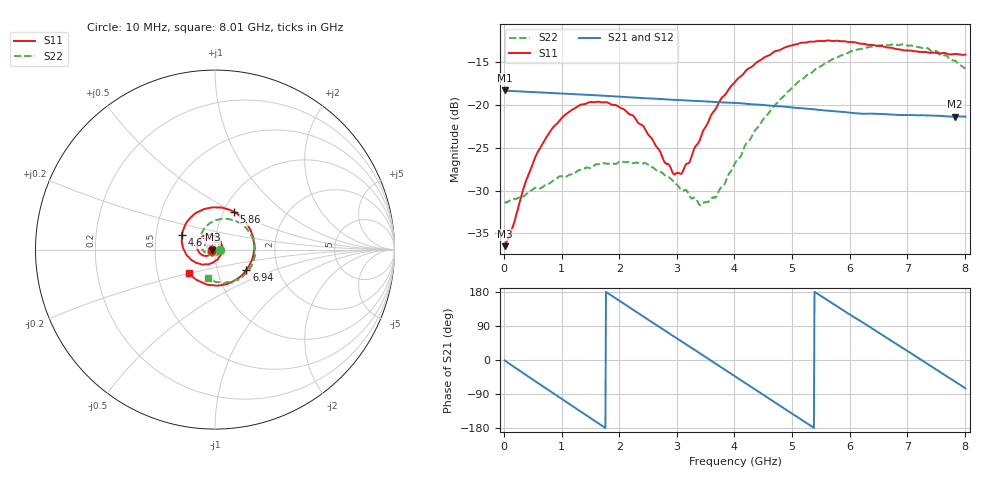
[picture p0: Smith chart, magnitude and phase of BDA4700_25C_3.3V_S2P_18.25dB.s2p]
!Agilent Technologies,E5071B,MY42404982,A.09.10
!Date: Mon Oct 20 18:10:42 2025
!Data & Calibration Information:
!Freq	S11:SOLT2(ON)	S21:SOLT2(ON)	S12:SOLT2(ON)	S22:SOLT2(ON)
# Hz S RI R 50
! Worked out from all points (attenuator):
!   801 points, 10 MHz to 8.01 GHz, reference 50 ohm
!   highest |S21| = -18.33 dB at 10 MHz (marker M1); lowest = -21.4 dB at 7.83 GHz (marker M2)
!   lowest |S11| = -36.5 dB at 10 MHz (marker M3), VSWR 1.03, Z = 48.5 - j0.122 ohm
!   |S11| at or under -10 dB: start of sweep to end of sweep
!   |S22| runs from -31.7 to -12.9 dB; largest |S21 - S12| = 0.0014
!   S11 on the Smith chart (normalised r, x): 10 MHz: 0.97, -0.00; 4.67 GHz: 0.68, +0.12; 5.86 GHz: 1.12, +0.50; 6.94 GHz: 1.38, -0.33; 8.01 GHz: 0.72, -0.20
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1e7  -0.0149 -0.00126  0.1212 -0.00264  0.1211 -0.00275  0.027 -0.000854
5.9e8  -0.0409 -0.0345  0.0576 -0.1033  0.0575 -0.1033  0.0135 -0.0298
1e9  -0.0799 -0.0244  -0.0253 -0.1136  -0.0252 -0.1138  -0.0158 -0.0349
1.35e9  -0.0999 0.0099  -0.0852 -0.0768  -0.0852 -0.0769  -0.0381 -0.0171
2.07e9  -0.0468 0.0819  -0.0959 0.0563  -0.096 0.0563  -0.029 0.0363
2.42e9  0.0029 0.0749  -0.0456 0.0994  -0.0457 0.0994  -0.00116 0.0455
2.68e9  0.0309 0.0458  0.00224 0.1082  0.00205 0.1081  0.0172 0.0371
2.94e9  0.0392 0.0056  0.0484 0.0953  0.0483 0.0951  0.0286 0.0213
3.08e9  0.0355 -0.0176  0.0698 0.0803  0.069 0.0807  0.0305 0.00948
3.4e9  0.00224 -0.0624  0.1001 0.0317  0.1002 0.0318  0.0214 -0.0149
3.54e9  -0.0212 -0.0759  0.1043 0.00674  0.1043 0.00655  0.0123 -0.0242
3.69e9  -0.0511 -0.0819  0.1017 -0.02  0.1018 -0.0203  -0.00134 -0.0293
4.01e9  -0.1186 -0.0659  0.075 -0.0699  0.0751 -0.0697  -0.0357 -0.028
4.67e9  -0.1843 0.0822  -0.0317 -0.0932  -0.0314 -0.0934  -0.0837 0.0489
5.35e9  -0.0557 0.2267  -0.0941 -0.00637  -0.094 -0.00703  -0.0139 0.1537
5.86e9  0.1071 0.2086  -0.0632 0.0653  -0.0632 0.0653  0.1054 0.1633
6.26e9  0.1972 0.1105  -0.00934 0.0881  -0.00809 0.088  0.1891 0.0996
6.68e9  0.2129 -0.0324  0.0505 0.072  0.0507 0.0719  0.2226 -0.00905
6.94e9  0.1747 -0.113  0.0754 0.0436  0.0756 0.0431  0.2098 -0.0809
7.41e9  0.038 -0.1974  0.0833 -0.0237  0.0833 -0.0238  0.1174 -0.1691
7.83e9  -0.0998 -0.171  0.0467 -0.0713  0.0467 -0.0715  0.00322 -0.1805
8.01e9  -0.1451 -0.1323  0.0223 -0.0823  0.0227 -0.0824  -0.039 -0.1572
